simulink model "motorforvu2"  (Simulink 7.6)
settings: Solver=ode45  StartTime=0.0  StopTime=inf  MaxStep=0.01  RelTol=1e-3
undefined symbols (not defined in the file or in its folder): settout

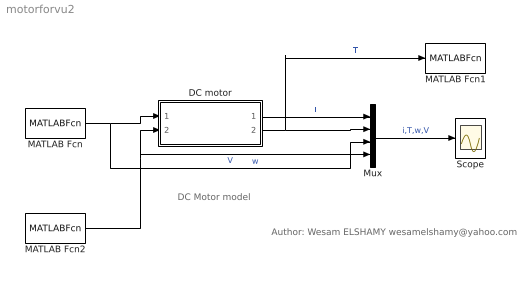
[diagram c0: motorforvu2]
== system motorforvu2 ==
  note: DC Motor model
  note: Author: Wesam ELSHAMY wesamelshamy@yahoo.com
  DC motor : Subsystem  mask(DC Motor){L=0.1, Kphi=0.3, J=1, b=0.01, R=2}
      mask help: Takes the DC voltage as input, and outputs angular velocity (w) and current (i) L => windings inductance Kphi => emf constant J => loads moment of inertial b => viscous friction R => windings resistance
  MATLAB Fcn : MATLABFcn  MATLABFcn=getvin  OutputSignalType=real
  MATLAB Fcn1 : MATLABFcn  MATLABFcn=settout(u)  OutputDimensions=0  OutputSignalType=real
  MATLAB Fcn2 : MATLABFcn  MATLABFcn=getwin  OutputSignalType=real
  Mux : Mux
  Scope : Scope
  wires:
  MATLAB Fcn/1 -> DC motor/1(V), Mux/3  "V"
  DC motor/1(i) -> Mux/1  "i"
  Mux/1 -> Scope/1  "i,T,w,V"
  DC motor/2(T) -> Mux/2, MATLAB Fcn1/1  "T"
  MATLAB Fcn2/1 -> DC motor/2(w), Mux/4  "w"

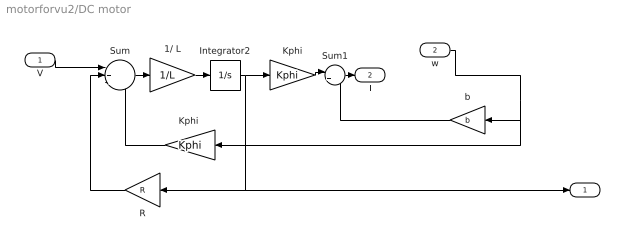
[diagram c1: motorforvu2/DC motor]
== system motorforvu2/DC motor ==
  note: i
  V : Inport
  w : Inport  Port=2
  1/ L : Gain  Gain=1/L
  Integrator2 : Integrator
  Kphi : Gain  Gain=Kphi
  "Kphi " : Gain  Gain=Kphi
  R : Gain  Gain=R
  Sum : Sum  Inputs=|+--
  Sum1 : Sum  Inputs=|+-
  b : Gain  Gain=b
  i : Outport
  T : Outport  Port=2
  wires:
  V/1 -> Sum/1
  Sum/1 -> 1/ L/1
  1/ L/1 -> Integrator2/1
  Integrator2/1 -> Kphi/1, R/1, i/1
  Kphi/1 -> Sum1/1
  Sum1/1 -> T/1
  w/1 -> "Kphi "/1, b/1
  b/1 -> Sum1/2
  "Kphi "/1 -> Sum/3
  R/1 -> Sum/2
